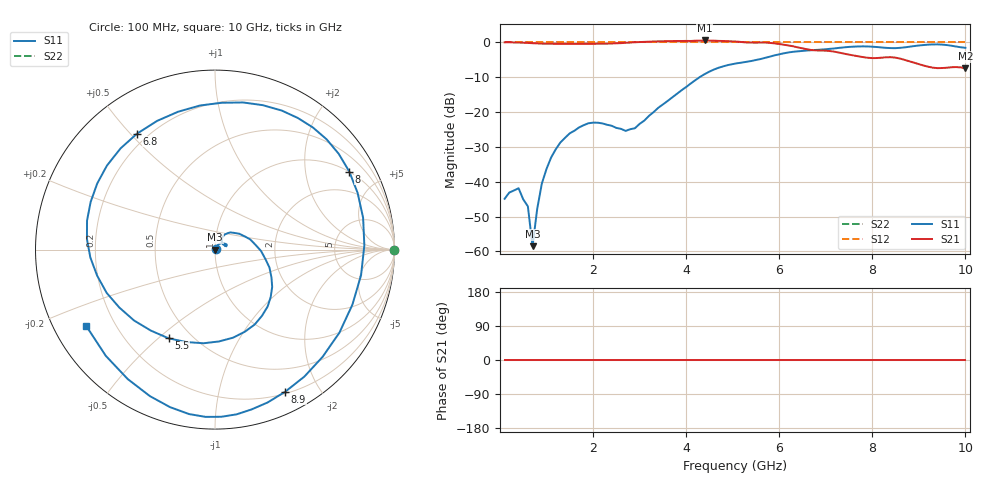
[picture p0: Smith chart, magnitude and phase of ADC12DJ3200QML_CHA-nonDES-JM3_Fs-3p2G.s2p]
!	Texas	"Instruments,"	Inc.
!	ADC12DJ3200	-	CH	A	S-Parameters	(nonDES	"Mode,"	Fs	=	3.2	"GSPS,"	25	degC	"case,"	15	degC	juntion)
!	Port	1	represents	the	100-ohm	differential	"input,"	Port	2	the	digital	output
!	freq	dbS11	angS11	dbS21	angS21	dbS12	angS12	dbS22	angS22
#	HZ	S	DB	R	100
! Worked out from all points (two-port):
!   100 points, 100 MHz to 10 GHz, reference 100 ohm
!   highest |S21| = 0.53 dB at 4.4 GHz (marker M1); lowest = -7.5 dB at 10 GHz (marker M2)
!   |S21| within 3 dB of the highest: start of sweep to 7.057 GHz
!   lowest |S11| = -58.5 dB at 700 MHz (marker M3), VSWR 1.00, Z = 100 - j0.149 ohm
!   |S11| at or under -10 dB: start of sweep to 4.29 GHz
!   |S22| runs from 0.0 to 0.0 dB; largest |S21 - S12| = 0.58
!   S11 on the Smith chart (normalised r, x): 100 MHz: 1.01, +0.00; 5.5 GHz: 0.38, -0.54; 6.8 GHz: 0.16, +0.52; 8 GHz: 0.99, +3.44; 8.9 GHz: 0.22, -1.59; 10 GHz: 0.10, -0.27
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1e8  -44.89 13.5  0.00 0.0  0.00 0.0  0.00 0.0
4e8  -41.86 -33.2  -0.07 0.0  0.00 0.0  0.00 0.0
6e8  -47.05 -42.4  -0.18 0.0  0.00 0.0  0.00 0.0
7e8  -58.48 -38.7  -0.26 0.0  0.00 0.0  0.00 0.0
9e8  -40.52 69.8  -0.37 0.0  0.00 0.0  0.00 0.0
1.1e9  -33.02 65.1  -0.42 0.0  0.00 0.0  0.00 0.0
1.8e9  -23.77 30.3  -0.43 0.0  0.00 0.0  0.00 0.0
2.7e9  -25.41 32.0  -0.14 0.0  0.00 0.0  0.00 0.0
3.4e9  -18.80 52.5  0.27 0.0  0.00 0.0  0.00 0.0
4.4e9  -9.11 -26.1  0.53 0.0  0.00 0.0  0.00 0.0
5.1e9  -6.00 -78.4  0.20 0.0  0.00 0.0  0.00 0.0
5.5e9  -5.07 -117.6  -0.09 0.0  0.00 0.0  0.00 0.0
6.1e9  -3.15 -176.4  -0.71 0.0  0.00 0.0  0.00 0.0
6.7e9  -2.26 133.0  -2.23 0.0  0.00 0.0  0.00 0.0
6.8e9  -2.18 123.9  -2.33 0.0  0.00 0.0  0.00 0.0
7.4e9  -1.44 71.7  -3.27 0.0  0.00 0.0  0.00 0.0
8e9  -1.26 30.2  -4.54 0.0  0.00 0.0  0.00 0.0
8.4e9  -1.66 -9.9  -4.27 0.0  0.00 0.0  0.00 0.0
8.9e9  -1.08 -63.7  -5.85 0.0  0.00 0.0  0.00 0.0
9.5e9  -0.65 -99.0  -7.38 0.0  0.00 0.0  0.00 0.0
9.8e9  -1.21 -124.0  -7.10 0.0  0.00 0.0  0.00 0.0
1e10  -1.58 -149.2  -7.47 0.0  0.00 0.0  0.00 0.0
